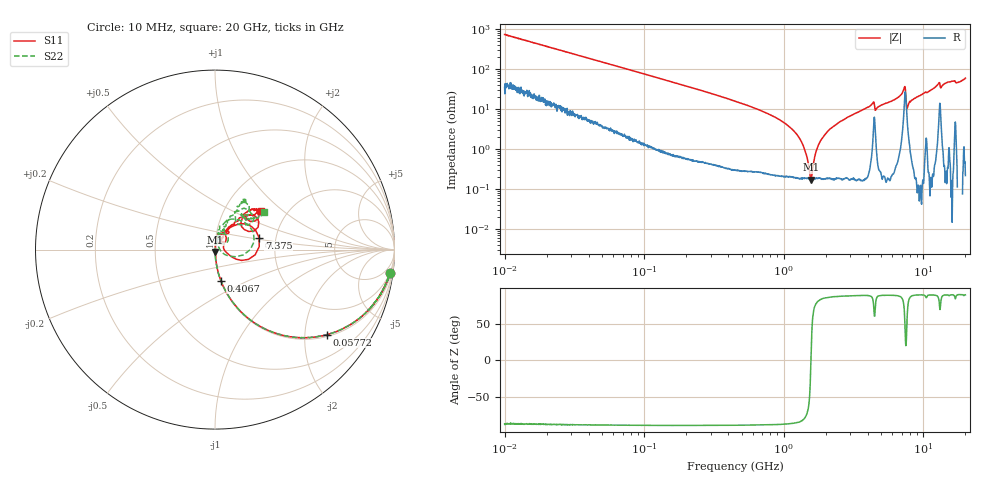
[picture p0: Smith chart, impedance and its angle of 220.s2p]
!Keysight Technologies,P5008B,MY61100088,A.16.20.02
!Date: Friday, August 30, 2024 13:48:35
!Correction: S11(C  2-Port  )
!S21(C  2-Port  )
!S12(C  2-Port  )
!S22(C  2-Port  )
!S2P File: Measurements: S11, S21, S12, S22:Log Frequency Sweep
# Hz S  MA  R 50
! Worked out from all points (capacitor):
!   1601 points, 10 MHz to 20 GHz, reference 50 ohm
!   read as one part in series: C = 21.7 pF near 10.39 MHz
!   lowest |Z| = 170 mohm at 1.567 GHz (marker M1)
!   series resonance near 1.565 GHz, so ESL is about 480 pH
!   S11 on the Smith chart (normalised r, x): 10 MHz: 2, -15; 57.72 MHz: 1.06, -2.59; 406.7 MHz: 1.00, -0.36; 7.375 GHz: 1.63, +0.23; 20 GHz: 1.49, +0.72
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1e7  0.9851 -7.7  0.1344 79.6  0.1344 79.6  0.9846 -7.7
3.555162e7  0.892 -25.3  0.4261 63.0  0.4261 63.0  0.892 -25.2
5.771651e7  0.7832 -37.2  0.6044 51.5  0.6042 51.5  0.783 -37.2
1.263918e8  0.5095 -58.7  0.8528 30.5  0.8526 30.5  0.5096 -58.7
4.066794e8  0.1758 -79.2  0.9814 9.7  0.9813 9.7  0.1759 -79.4
4.472136e8  0.1589 -80.2  0.9845 8.7  0.9841 8.7  0.1588 -80.5
1.007657e9  0.05357 -85.3  0.9966 2.1  0.9964 2.1  0.05347 -86.5
1.567418e9  0.01362 -80.2  0.9982 -0.8  0.9981 -0.8  0.01364 -87.5
1.589917e9  0.01247 -80.3  0.9982 -0.9  0.998 -0.9  0.01256 -86.2
1.707346e9  0.006426 -77.6  0.9983 -1.3  0.9981 -1.4  0.006648 -72.7
1.798938e9  0.00364 -31.9  0.9982 -1.7  0.9981 -1.7  0.001953 -72.4
1.859765e9  0.004185 8.7  0.9983 -1.9  0.9983 -1.9  0.0006626 139.6
2.074486e9  0.009497 76.9  0.9984 -2.7  0.9982 -2.7  0.009193 73.7
2.449743e9  0.02159 86.2  0.9983 -3.9  0.9981 -3.9  0.02136 74.8
4.291128e9  0.08817 76.5  0.9883 -10.1  0.9878 -10.1  0.08921 71.8
4.652055e9  0.05582 80.5  0.9927 -8.9  0.9924 -8.9  0.05781 68.7
5.652411e9  0.07865 76.1  0.9965 -12.4  0.9962 -12.5  0.08169 74.8
7.167884e9  0.1934 47.0  0.9444 -20.4  0.9442 -20.5  0.1842 65.2
7.375132e9  0.2545 15.2  0.8029 -19.2  0.803 -19.3  0.2343 23.8
7.91985e9  0.06257 34.4  0.9875 -13.9  0.9873 -14.1  0.04824 85.1
1.261552e10  0.2477 48.9  0.9633 -31.2  0.963 -31.4  0.2436 60.5
2e10  0.3356 39.6  0.9427 -50.9  0.9425 -51.2  0.3427 37.5
